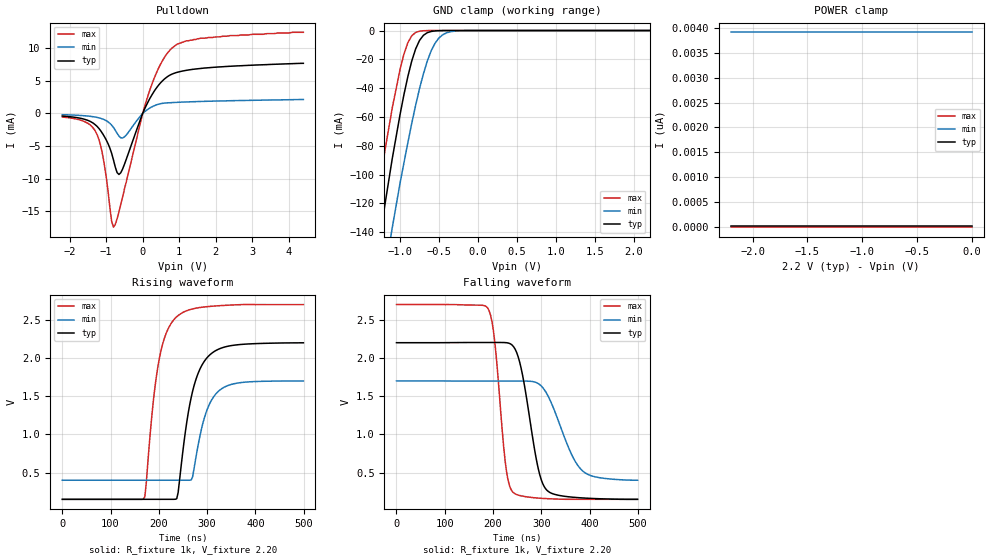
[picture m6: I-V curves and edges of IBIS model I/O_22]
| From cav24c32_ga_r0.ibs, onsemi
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[Model] I/O_22
Model_type I/O_open_drain
Vinh =  1.54
Vinl =  0.66
Vmeas = 1.10
Vref = 2.20
Rref = 1000
Cref = 0pF
|  variable   typ   min   max
C_comp   8.00pF   NA   8.00pF
|//////////////////////////////////////////////////////////////////////////////
[Temperature Range]   25   NA   -40
|//////////////////////////////////////////////////////////////////////////////
[Voltage Range]   2.20V   NA   2.70V
|//////////////////////////////////////////////////////////////////////////////
[Pulldown Reference]   0V   NA   0V
|//////////////////////////////////////////////////////////////////////////////
[POWER Clamp Reference] 2.20V   NA   2.70V
|////////////////////////////////////////////////////////////////////////
[GND Clamp Reference]   0V   NA   0V
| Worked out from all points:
|   slope of the pulldown table from 0 to 0.33 V, typ, clamps not added: 94 ohm
|   GND clamp passes 1 mA (typ) near -0.62 V on its own axis
|   falling waveform, R_fixture 1k, V_fixture 2.20: 20-80 % time 32.7ns typ, 50.4ns min, 21ns max; typ from 2.2 V to 0.15 V
|   rising waveform, R_fixture 1k, V_fixture 2.20: 20-80 % time 35.1ns typ, 32.6ns min, 30.6ns max; typ from 0.15 V to 2.2 V
|//////////////////////////////////////////////////////////////////////////////
[Pulldown]
|   Voltage   I(typ)   I(min)   I(max)
-2.2V     -408uA     -200uA     -558uA
-1.6V     -885uA     -357uA     -1.23mA
-1.25V    -1.98mA    -615uA     -3.22mA
-1.1V     -3.07mA    -851uA     -6.24mA
-850mV    -6.1mA     -1.79mA    -16.5mA
-800mV    -7.11mA    -2.14mA    -17.4mA
-700mV    -9.06mA    -3.04mA    -16.1mA
-600mV    -9.08mA    -3.73mA    -13.9mA
150mV     1.79mA     659uA      2.8mA
750mV     5.87mA     1.63mA     9.7mA
1.6V      6.88mA     1.83mA     11.5mA
4.4V      7.66mA     2.12mA     12.4mA
|//////////////////////////////////////////////////////////////////////////////
[GND Clamp]
|   Voltage   I(typ)   I(min)   I(max)
-2.2V     -961mA     -980mA     -956mA
-1.4V     -228mA     -270mA     -203mA
-1.3V     -165mA     -211mA     -130mA
-1.2V     -123mA     -170mA     -85.3mA
-1.1V     -89mA      -137mA     -53.8mA
-950mV    -44.5mA    -91.9mA    -16.4mA
-900mV    -32mA      -77.9mA    -8.5mA
-800mV    -12.8mA    -51.9mA    -1.35mA
-700mV    -3.31mA    -30mA      -151uA
-600mV    -634uA     -14mA      -15.8uA
-400mV    -18.9uA    -1.53mA    -172nA
2.2V      22pA       3.91nA     82.6fA
|//////////////////////////////////////////////////////////////////////////////
[POWER Clamp]
|   Voltage   I(typ)   I(min)   I(max)
-2.2V     22pA       3.91nA     82.6fA
-2.1V     22pA       3.91nA     82.6fA
-2V       22pA       3.91nA     82.6fA
0V        22pA       3.91nA     82.6fA
|//////////////////////////////////////////////////////////////////////////////
|//////////////////////////////////////////////////////////////////////////////
[Ramp]
|  variable   typ   min   max
dV/dt_r   1.230E+00/3.600E-08  9.510E-01/3.300E-08  1.530E+00/3.000E-08
dV/dt_f   1.230E+00/3.300E-08  9.510E-01/5.100E-08  1.530E+00/2.100E-08
R_load = 1k
|/////////////////////////////////////////////////////////////////////////////
[Falling Waveform]
R_fixture = 1k
V_fixture = 2.20
V_fixture_min = 1.70
V_fixture_max = 2.70
C_fixture = 0p
|   time   V(typ)   V(min)   V(max)
0s        2.2V       1.7V       2.7V
189ns     2.203V     1.698V     2.653V
204ns     2.203V     1.698V     2.193V
228ns     2.2V       1.698V     514.7mV
243ns     2.145V     1.697V     233.8mV
261ns     1.784V     1.697V     192.3mV
294ns     545.1mV    1.664V     166mV
309ns     288.5mV    1.559V     159.8mV
384ns     168.9mV    532.1mV    150mV
499.5ns   150mV      400mV      150mV
|//////////////////////////////////////////////////////////////////////////////
[Rising Waveform]
R_fixture = 1k
V_fixture = 2.20
V_fixture_min = 1.70
V_fixture_max = 2.70
C_fixture = 0p
|   time   V(typ)   V(min)   V(max)
0s        150mV      400mV      150mV
168ns     150mV      400mV      151.8mV
174ns     150mV      400mV      368mV
189ns     150mV      400mV      1.461V
201ns     150mV      400mV      1.993V
240ns     238.4mV    400mV      2.557V
267ns     1.483V     403.5mV    2.639V
300ns     2.005V     1.324V     2.673V
348ns     2.161V     1.651V     2.694V
499.5ns   2.2V       1.7V       2.7V
